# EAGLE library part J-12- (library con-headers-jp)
HEADER JACK PINS
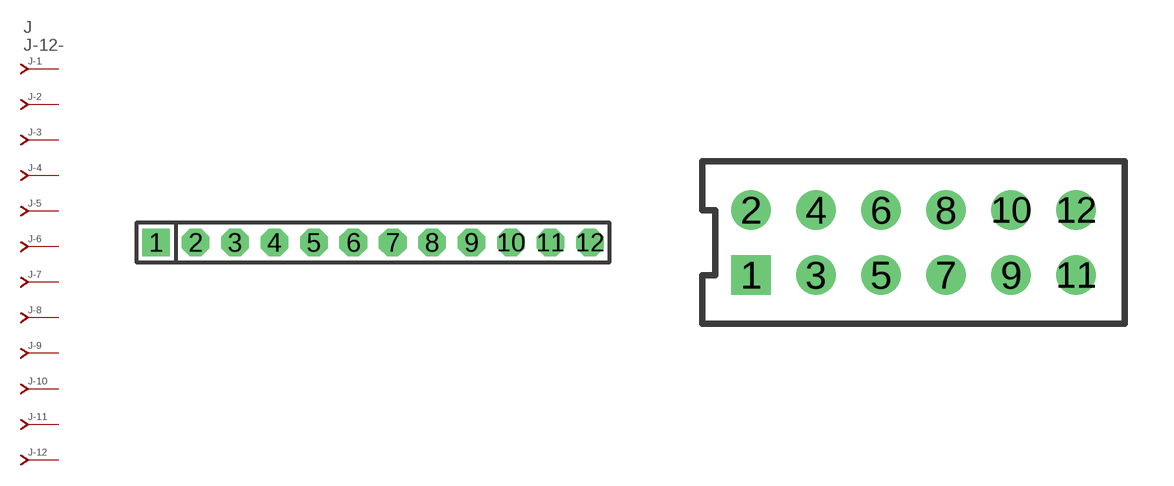
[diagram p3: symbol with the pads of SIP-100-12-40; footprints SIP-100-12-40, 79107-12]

Designator prefix J; gates -2=J-N -3=J-N -4=J-N -5=J-N -6=J-N -7=J-N -8=J-N -9=J-N -10=J-N -11=J-N -12=J-N -1=J-NV

## J-12-SIP-100-40  [SIP-100-12-40]
1  -1:J  pas
2  -2:J  pas
3  -3:J  pas
4  -4:J  pas
5  -5:J  pas
6  -6:J  pas
7  -7:J  pas
8  -8:J  pas
9  -9:J  pas
10  -10:J  pas
11  -11:J  pas
12  -12:J  pas

## J-12-79107  [79107-12]
Pads as for SIP-100-12-40

## J-12-79109  [79109-12]
Pads as for SIP-100-12-40

## J-12-87264  [87264-12]
Pads as for SIP-100-12-40

## J-12-87368  [87368-12]
Pads as for SIP-100-12-40

## J-12-87340  [87340-12]
Pads as for SIP-100-12-40

## J-12-535512  [535512-12]
Pads as for SIP-100-12-40

## J-12-100-2X06  [DIL-100-2X06]
Pads as for SIP-100-12-40

## J-12-100-2X06_M  [DIL-100-2X06_M]
Pads as for SIP-100-12-40

## J-12-2MM-2X06  [DIL-2MM-2X06]
Pads as for SIP-100-12-40

## J-12-2MM-2X06_M  [DIL-2MM-2X06_M]
Pads as for SIP-100-12-40

## J-12-SIP-100-32  [SIP-100-12-32]
Pads as for SIP-100-12-40

## J-12-SIP-100-40Y  [SIP-100-12-40Y]
Pads as for SIP-100-12-40

## J-12-SIP-100-32Y  [SIP-100-12-32Y]
Pads as for SIP-100-12-40

## J-12-71991  [71991-12]
Pads as for SIP-100-12-40

## J-12-KK-4455-B12  [KK-4455-B12]
Pads as for SIP-100-12-40

## J-12-KK-4455-A12  [KK-4455-A12]
Pads as for SIP-100-12-40

## J-12-KK-4455-C12  [KK-4455-C12]
Pads as for SIP-100-12-40

## Footprint SIP-100-12-40 (pad centres in mm)
SIP Header - 0.1", 40 mil drill
drill 1.016 pad 1.778 square: 1 -13.97,0
drill 1.016 pad 1.778 octagon: 2 -11.43,0; 3 -8.89,0; 4 -6.35,0; 5 -3.81,0; 6 -1.27,0; 7 1.27,0; 8 3.81,0; 9 6.35,0; 10 8.89,0; 11 11.43,0; 12 13.97,0

## Footprint 79107-12 (pad centres in mm)
Molex Board-To-Board Receptacal 2.00mm (.079") Pitch Milli-Grid Header, Vertical, Through-Hole Mates with: 87759, 87762, 87758, 87760
drill 0.711 square: 1 -5,-1
drill 0.711: 2 -5,1; 3 -3,-1; 4 -3,1; 5 -1,-1; 6 -1,1; 7 1,-1; 8 1,1; 9 3,-1; 10 3,1; 11 5,-1; 12 5,1

## Footprint 79109-12 (pad centres in mm)
Molex Board-to-Board Receptacal 2.00mm (.079") Pitch Milli-Grid Header, Vertical, Top/Bottom Entry Mates with: 87758, 87759, 87760, 87831, 87832, 87833
smd 1.12 x 1.83: 1 -5,-2.65; 2 -5,2.65; 3 -3,-2.65; 4 -3,2.65; 5 -1,-2.65; 6 -1,2.65; 7 1,-2.65; 8 1,2.65; 9 3,-2.65; 10 3,2.65; 11 5,-2.65; 12 5,2.65
hole 0.914 at -4,0
hole 0.914 at -5,1
hole 0.914 at -5,-1
hole 0.914 at -3,-1
hole 0.914 at -3,1
hole 0.914 at -1,-1
hole 0.914 at -1,1
hole 0.914 at 4,0
hole 0.914 at 1,1
hole 0.914 at 1,-1
hole 0.914 at 3,1
hole 0.914 at 3,-1
hole 0.914 at 5,1
hole 0.914 at 5,-1

## Footprint 87264-12 (pad centres in mm)
Molex Board-To-Board Receptacal 2.00mm (.079") Pitch Milli-Grid Header, Side Entry Mates with 2mm(.079") Mill-Grid Header
drill 0.914 square: 1 -5,-2.25
drill 0.914: 2 -5,2.25; 3 -3,-2.25; 4 -3,2.25; 5 -1,-2.25; 6 -1,2.25; 7 1,-2.25; 8 1,2.25; 9 3,-2.25; 10 3,2.25; 11 5,-2.25; 12 5,2.25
